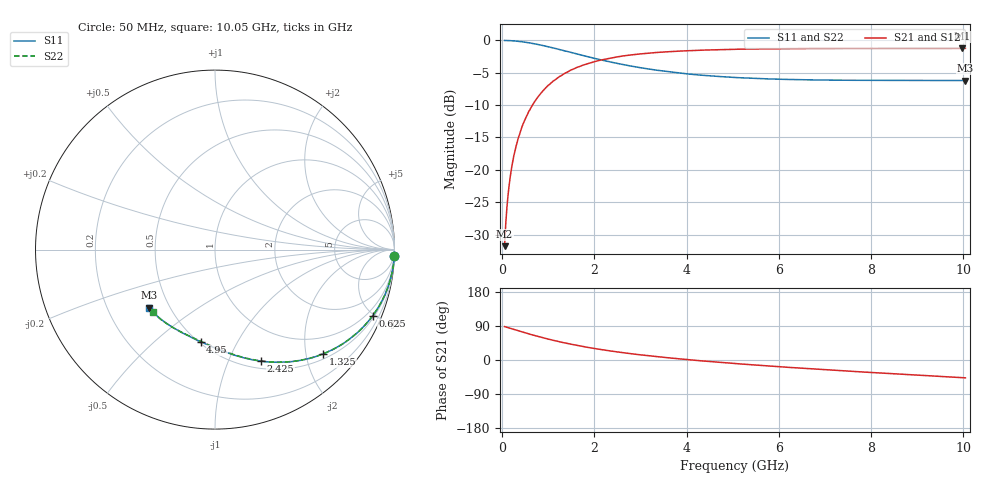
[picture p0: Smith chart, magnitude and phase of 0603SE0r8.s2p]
! AVX Thin Film Operation		Date: August 2001
! Description: Accu-P® Series, Thin Film, SMD, RF Capacitor
! Part Number: 06035J0R8ABT
! 50 MHz  -  10.05 GHz
! Serial Measurements
# mhz S db R 50
!	S11		S21		S12		S22
!	dB	Phase	dB	Phase	dB	Phase	dB	Phase
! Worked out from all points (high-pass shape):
!   401 points, 50 MHz to 10.05 GHz, reference 50 ohm
!   highest |S21| = -1.22 dB at 9.975 GHz (marker M1); lowest = -31.8 dB at 50 MHz (marker M2)
!   |S21| within 3 dB of the highest: 1.605 GHz to end of sweep
!   lowest |S11| = -6.2 dB at 10.05 GHz (marker M3), VSWR 2.92, Z = 19.2 - j16.3 ohm
!   |S11| at or under -10 dB: nowhere
!   |S22| runs from -6.2 to 0.0 dB; largest |S21 - S12| = 0
!   S11 on the Smith chart (normalised r, x): 50 MHz: 1, -61; 625 MHz: 0.61, -4.87; 1.325 GHz: 0.61, -2.34; 2.425 GHz: 0.58, -1.33; 4.95 GHz: 0.51, -0.72; 10.05 GHz: 0.38, -0.33
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50  -0.00 -1.9  -31.80 88.1  -31.80 88.1  -0.00 -1.9
75  -0.01 -2.8  -28.31 87.2  -28.31 87.2  -0.01 -2.8
150  -0.03 -5.6  -22.31 84.4  -22.31 84.4  -0.03 -5.6
200  -0.05 -7.5  -19.79 82.5  -19.79 82.5  -0.05 -7.5
250  -0.07 -9.4  -17.84 80.6  -17.84 80.6  -0.07 -9.4
300  -0.10 -11.2  -16.33 78.8  -16.33 78.8  -0.10 -11.2
400  -0.18 -14.9  -13.93 75.1  -13.93 75.1  -0.18 -14.9
500  -0.28 -18.5  -12.11 71.5  -12.11 71.5  -0.28 -18.5
625  -0.42 -22.9  -10.35 67.2  -10.35 67.2  -0.42 -22.8
950  -0.90 -33.4  -7.28 56.6  -7.28 56.6  -0.90 -33.4
1325  -1.56 -44.1  -5.22 45.9  -5.22 45.9  -1.56 -44.0
1725  -2.29 -53.8  -3.89 36.2  -3.89 36.2  -2.29 -53.8
2425  -3.44 -67.5  -2.62 22.5  -2.62 22.5  -3.44 -67.3
2900  -4.10 -75.0  -2.15 15.0  -2.15 15.0  -4.10 -74.8
3400  -4.64 -81.8  -1.84 8.3  -1.84 8.3  -4.64 -81.3
4125  -5.25 -90.4  -1.55 -0.2  -1.55 -0.2  -5.24 -89.7
4950  -5.69 -98.9  -1.39 -8.4  -1.39 -8.4  -5.68 -97.7
5050  -5.73 -99.7  -1.37 -9.4  -1.37 -9.4  -5.72 -98.6
6725  -6.10 -114.0  -1.25 -23.5  -1.25 -23.5  -6.08 -112.0
8400  -6.17 -127.2  -1.23 -35.8  -1.23 -35.8  -6.15 -124.2
9975  -6.19 -138.2  -1.22 -46.6  -1.22 -46.6  -6.17 -134.2
10050  -6.19 -138.8  -1.22 -47.1  -1.22 -47.1  -6.17 -134.8
